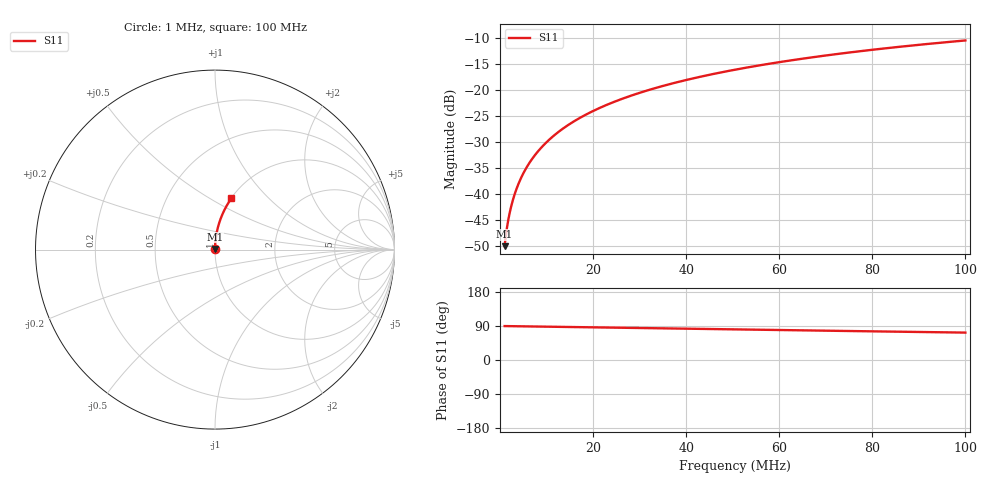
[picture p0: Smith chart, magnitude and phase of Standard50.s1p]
# MHz S RI R 50.0
! SimSmith 18.4g
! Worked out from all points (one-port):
!   1000 points, 1 MHz to 100 MHz, reference 50 ohm
!   lowest |S11| = -50.1 dB at 1 MHz (marker M1), VSWR 1.01, Z = 50 + j0.314 ohm
!   |S11| at or under -10 dB: start of sweep to end of sweep
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1  2.56e-05 0.00314
1.297297  3.7e-05 0.00408
1.693694  5.49e-05 0.00532
1.990991  7.04e-05 0.00625
2.387387  9.37e-05 0.0075
2.783784  0.00012 0.00874
3.279279  0.000158 0.0103
3.774775  0.0002 0.0119
4.369369  0.000257 0.0137
5.063063  0.000332 0.0159
5.855856  0.00043 0.0184
6.648649  0.00054 0.0209
7.54054  0.000679 0.0237
8.531531  0.000852 0.0268
10.81081  0.00132 0.0339
13.38739  0.00197 0.042
15.96396  0.00276 0.05
18.93694  0.00382 0.0592
22.20721  0.00519 0.0694
25.77478  0.00691 0.0804
31.52252  0.0102 0.098
38.16216  0.0147 0.1181
44.10811  0.0195 0.1358
50.54955  0.0253 0.1547
62.93694  0.0385 0.1899
75.32432  0.054 0.2236
87.71171  0.0717 0.2555
100  0.091 0.2851
